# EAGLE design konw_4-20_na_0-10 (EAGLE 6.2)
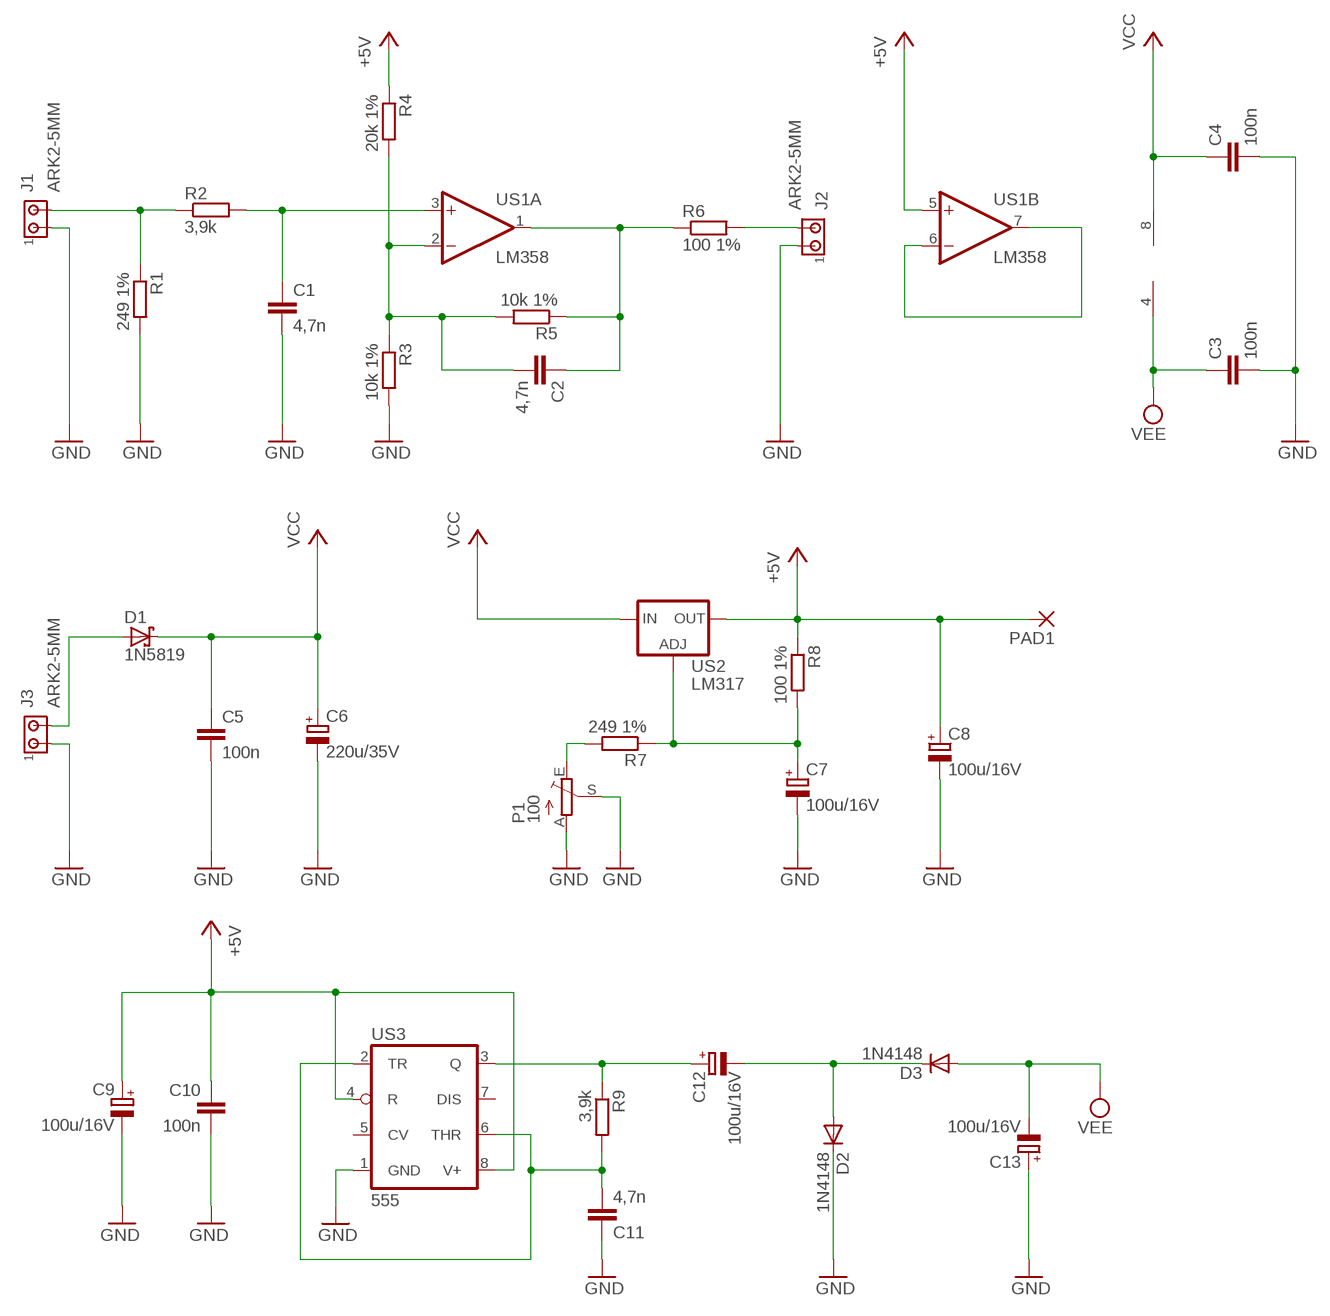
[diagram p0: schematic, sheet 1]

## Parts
C1  4,7n  C-EU050-025X075  [C050-025X075]
C2  4,7n  C-EU050-025X075  [C050-025X075]
C3  100n  C-EU050-025X075  [C050-025X075]
C4  100n  C-EU050-025X075  [C050-025X075]
C5  100n  C-EU050-025X075  [C050-025X075]
C6  220u/35V  CPOL-EUE3.5-8  [E3,5-8]
C7  100u/16V  CPOL-EUE2.5-6  [E2,5-6]
C8  100u/16V  CPOL-EUE2.5-6  [E2,5-6]
C9  100u/16V  CPOL-EUE2.5-6  [E2,5-6]
C10  100n  C-EU050-025X075  [C050-025X075]
C11  4,7n  C-EU050-025X075  [C050-025X075]
C12  100u/16V  CPOL-EUE2.5-6  [E2,5-6]
C13  100u/16V  CPOL-EUE2.5-6  [E2,5-6]
D1  1N5819  1N5819-T  [DO41-7.6]
D2  1N4148  BAT81  [DO34-7]
D3  1N4148  BAT81  [DO34-7]
J1  ARK2-5MM  [2PIN-5MM]
J2  ARK2-5MM  [2PIN-5MM]
J3  ARK2-5MM  [2PIN-5MM]
P1  100  TRIM_EU-B64Y  [B64Y]
PAD1  2,15/1,0  [2,15/1,0]
R1  249 1%  R-EU_0207/7  [0207/7]
R2  3,9k  R-EU_0207/7  [0207/7]
R3  10k 1%  R-EU_0207/7  [0207/7]
R4  20k 1%  R-EU_0207/7  [0207/7]
R5  10k 1%  R-EU_0207/7  [0207/7]
R6  100 1%  R-EU_0207/7  [0207/7]
R7  249 1%  R-EU_0207/7  [0207/7]
R8  100 1%  R-EU_0207/7  [0207/7]
R9  3,9k  R-EU_0207/7  [0207/7]
US1  LM358  LM358N  [DIL08]
US2  LM317  LM317TS  [317TS]
US3  555  LM555N  [DIL08]

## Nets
+5V: C8.+ C9.+ C10.1 PAD1.1(P) R4.1 R8.1 US1.5(B:+IN) US2.2(OUT) US3.4(R) US3.8(V+)
GND: C1.2 C3.2 C4.2 C5.2 C6.- C7.- C8.- C9.- C10.2 C11.1 C13.+ D2.C J1.P$1 J2.P$1 J3.P$1 P1.A P1.S R1.2 R3.2 US3.1(GND)
N$1: J1.P$2 R1.1 R2.1
N$2: C1.1 R2.2 US1.3(A:+IN)
N$3: C2.1 R5.1 R6.1 US1.1(A:OUT)
N$4: C2.2 R3.1 R4.2 R5.2 US1.2(A:-IN)
N$5: J2.P$2 R6.2
N$6: P1.E R7.2
N$9: US1.6(B:-IN) US1.7(B:OUT)
N$15: C12.- D2.A D3.C
N$16: C11.2 R9.2 US3.2(TR) US3.6(THR)
N$18: D1.A J3.P$2
N$19: C12.+ R9.1 US3.3(Q)
N$22: C7.+ R7.1 R8.2 US2.1(ADJ)
VCC: C4.1 C5.1 C6.+ D1.C US1.8(P:V+) US2.3(IN)
VEE: C3.1 C13.- D3.A US1.4(P:V-)
Unconnected: US3.5(CV) US3.7(DIS)

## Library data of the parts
C1-C5 C10 C11 = rcl:C-EU: CAPACITOR, European symbol
C6-C9 C12 C13 = rcl:CPOL-EU: POLARIZED CAPACITOR, European symbol
D1 = diode:1N581*: 1.0A SCHOTTKY BARRIER RECTIFIER
D2 D3 = diode:BAT81: DIODE
J1-J3 = zlacza_futrzak:ARK2: ARK 2
P1 = pot:TRIM_EU-: POTENTIOMETER
PAD1 = wirepad:2,15/1,0: THROUGH-HOLE PAD
R1-R9 = rcl:R-EU_: RESISTOR, European symbol
US1 = linear:LM358: OP AMP also LM158; LM258; LM2904 Source: http://cache.national.com/ds/LM/LM158.pdf
US2 = v-reg:LM317TS: VOLTAGE REGULATOR
US3 = linear:*555: TIMER

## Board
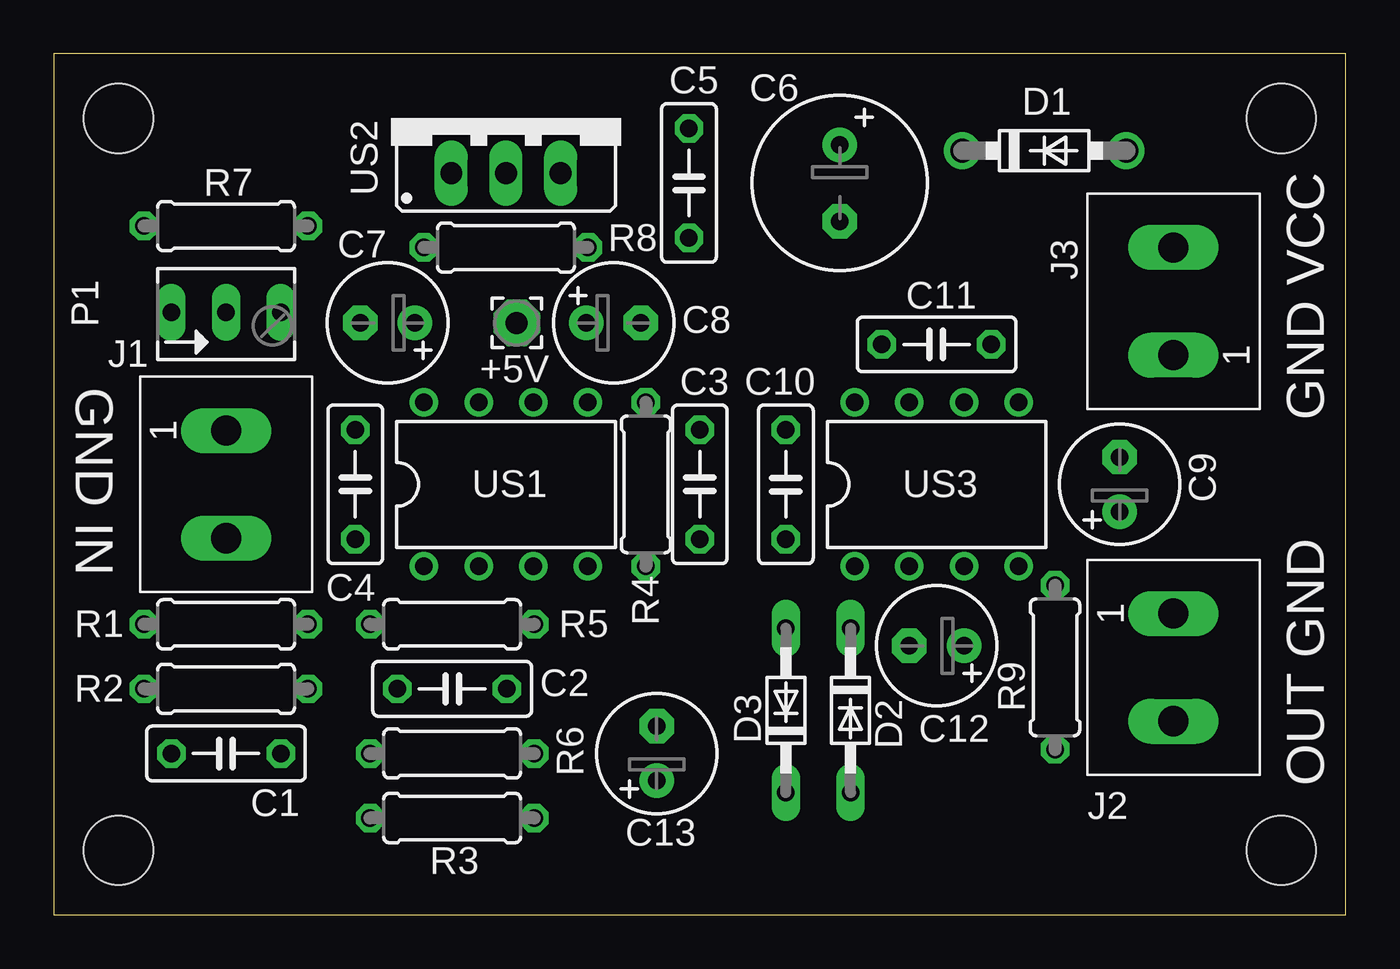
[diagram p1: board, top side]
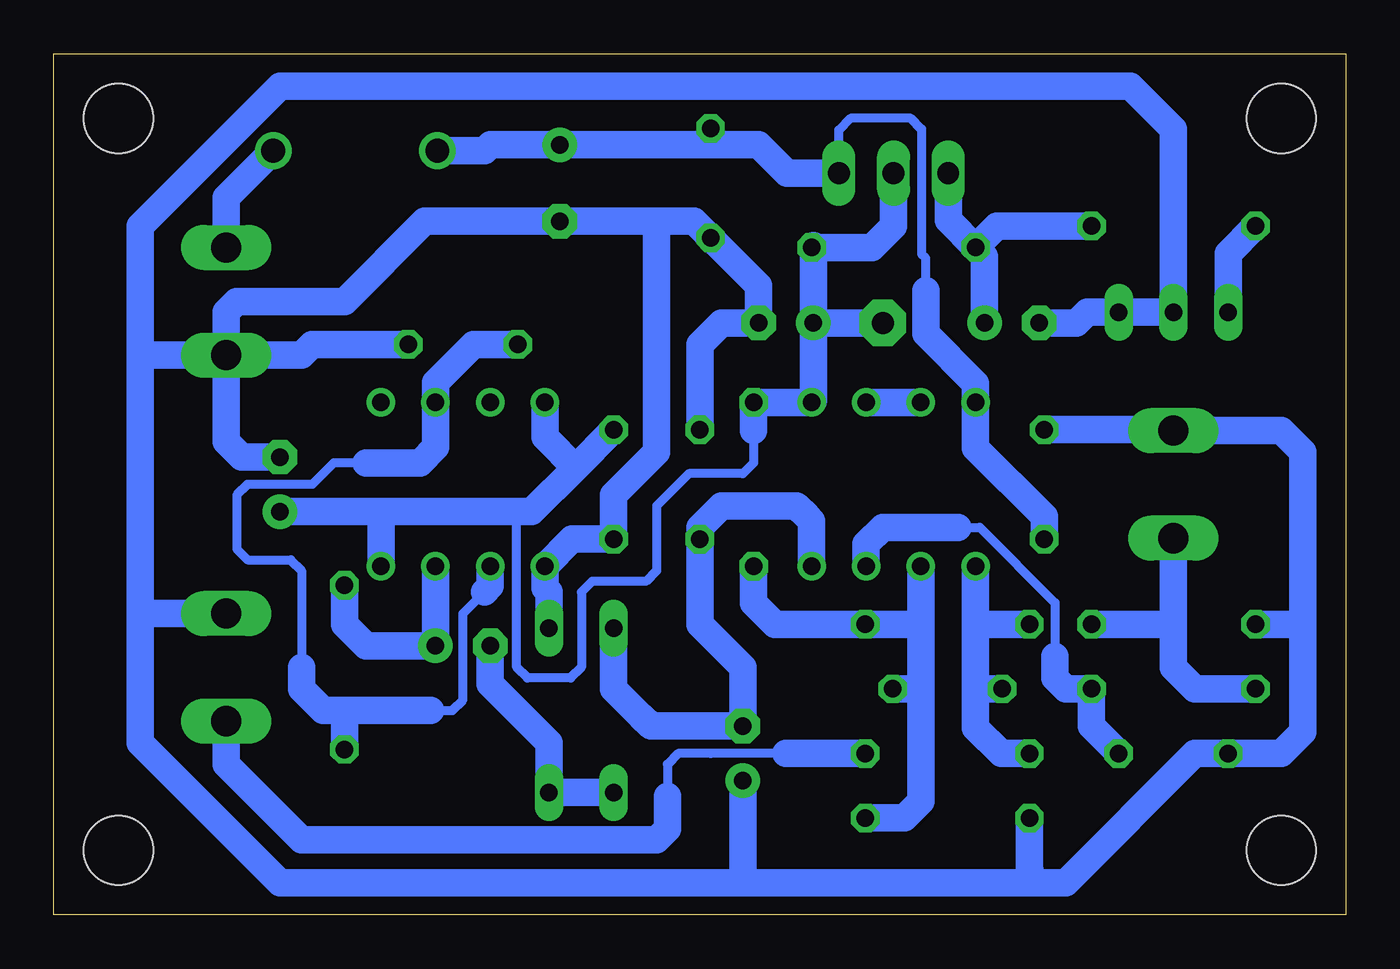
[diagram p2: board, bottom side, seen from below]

Size 60 x 40 mm. Coordinates in mm from the lower left corner, seen from the top.
Outline: 0,0 60,0 60,40 0,40 0,0
Copper layers (1*16): Top 0.035mm / dielectric 1.5mm / Bottom 0.035mm
Design rules: minimum track width 10mil, minimum drill 24mil, track to track 8mil, track to pad 8mil, pad to pad 8mil, via to via 8mil, smd to smd 8mil, copper to edge 20mil, drill to drill 8mil, minimum pad ring 10mil, minimum via ring 8mil, stop-mask expansion 4mil, vias tented up to drill 0mil, thermal gap 10mil
Holes 3.2 mm at 3,3 3,37 57,3 57,37

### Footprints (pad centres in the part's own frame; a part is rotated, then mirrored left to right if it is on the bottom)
C050-025X075 = drill 0.813 octagon: 1 -2.54,0; 2 2.54,0
E3,5-8 = drill 0.813 pad 1.6: + -1.778,0 | drill 0.813 pad 1.6 octagon: - 1.778,0
E2,5-6 = drill 0.813 pad 1.6: + -1.27,0 | drill 0.813 pad 1.6 octagon: - 1.27,0
DO41-7.6 = drill 1.1 pad 1.7: A 3.81,0; C -3.81,0
DO34-7 = drill 0.813 long: A 3.81,0; C -3.81,0
2PIN-5MM = drill 1.4 long: P$1 -2.5,0; P$2 2.5,0
B64Y = drill 0.813 long: A 2.54,0; E -2.54,0; S 0,0
2,15/1,0 = drill 1.016 pad 2.159 octagon: 1 0,0
0207/7 = drill 0.813 octagon: 1 -3.81,0; 2 3.81,0
DIL08 = drill 0.813 pad 1.27: 1 -3.81,-3.81; 2 -1.27,-3.81; 3 1.27,-3.81; 4 3.81,-3.81; 5 3.81,3.81; 6 1.27,3.81; 7 -1.27,3.81; 8 -3.81,3.81
317TS = drill 1.016 long: 1 -2.54,-2.54; 2 0,-2.54; 3 2.54,-2.54

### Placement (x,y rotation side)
C1  8,7.5 180 top
C2  18.5,10.5 0 top
C3  30,20 90 top
C4  14,20 90 top
C5  29.5,34 270 top
C6  36.5,34 270 top
C7  15.5,27.5 180 top
C8  26,27.5 0 top
C9  49.5,20 90 top
C10  34,20 270 top
C11  41,26.5 180 top
C12  41,12.5 180 top
C13  28,7.5 90 top
D1  46,35.5 0 top
D2  37,9.5 270 top
D3  34,9.5 90 top
J1  8,20 270 top
J2  52,11.5 270 top
J3  52,28.5 90 top
P1  8,28 0 top
PAD1  21.5,27.5 0 top
R1  8,13.5 180 top
R2  8,10.5 0 top
R3  18.5,4.5 180 top
R4  27.5,20 270 top
R5  18.5,13.5 0 top
R6  18.5,7.5 0 top
R7  8,32 180 top
R8  21,31 180 top
R9  46.5,11.5 270 top
US1  21,20 0 top
US2  21,37 0 top
US3  41,20 0 top

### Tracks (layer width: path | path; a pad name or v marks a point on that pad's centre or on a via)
+5V
  Bottom 0.406: 27.5,22.5 27.5,21 28,20.5 30.5,20.5 32,19 32,16 32.5,15.5 35,15.5 35.5,15 35.5,11.5 36,11 38,11 38.5,11.5 38.5,18.73
  Bottom 1.27: C9.+ 45,18.73 | 45,18.73 38.5,18.73 37.81,18.73 35.77,20.77 | 35.77,20.77 C10.1 | US3.8 37.19,22.19 35.77,20.77 | US3.4 44.81,18.54 45,18.73 | C8.+ 24.73,23.89 US1.5 R4.1 27.5,22.5 | C8.+ 24.73,31.08 R8.1 22,31 21,32 US2.2 | PAD1.1 C8.+
GND
  Bottom 1.27: 2,13.5 2,21.5 3,22.5 J1.P$1 8.04,22.54 C4.2 | 2,13.5 2,8.5 3,7.5 C1.2 7,7.5 13,1.5 14.5,1.5 | R1.2 2,13.5 | 14.5,1.5 28,1.5 | 28,1.5 49.5,1.5 56,8 56,14 | 56,14 56,26 | J3.P$1 56,26 | J2.P$1 56,14 | R3.2 14.69,2.19 14.5,1.5 | C13.+ 28,1.5 | D2.C 37,15 37.19,15.19 US3.1 35.92,17.46 C10.2 34,19.5 32,21.5 32,32.22 | 56,26 56,32 49.5,38.5 10,38.5 8,36.5 P1.S P1.A 12,28 12.5,27.5 C7.- | C11.1 48,26.5 48.5,26 J3.P$1 | J3.P$1 52,22 51.27,21.27 C9.- | J3.P$1 52,28 51.5,28.5 46.5,28.5 42.78,32.22 C6.- 32,32.22 | 32,32.22 30.26,32.22 C5.2 27.27,29.23 C8.- 29,27.5 30,26.5 C3.2
N$1
  Bottom 1.27: J1.P$2 8,13.5 | 8,13.5 8,11.5 7,10.5 R2.1 | R1.1 8,13.5
N$2
  Bottom 0.406: 18,18 17,18 13.5,14.5 13.5,12
  Bottom 1.27: C1.1 11.81,8.77 R2.2 13,10.5 13.5,11 13.5,12 | US1.3 22.27,17.23 21.5,18 18,18
N$3
  Bottom 1.27: US1.1 17.19,13.5 | 17.19,13.5 17.19,10.5 | 17.19,10.5 17.19,8.69 16,7.5 R6.1 | C2.1 17.19,10.5 | R5.1 17.19,13.5
N$4
  Bottom 1.27: US1.2 19.73,13.5 | 19.73,13.5 19.73,10.5 | 19.73,10.5 19.73,5.27 20.5,4.5 R3.1 | C2.2 19.73,10.5 | 19.73,13.5 R5.2 26.5,13.5 27.5,14.5 R4.2
N$5
  Bottom 0.406: 26,7.5 29.5,7.5 31,7.5 31.5,7 31.5,5.5
  Bottom 1.27: R6.2 26,7.5 | 31.5,5.5 31.5,4 32,3.5 48.5,3.5 52,7 J2.P$2
N$6
  Bottom 1.27: P1.E 5.46,30.73 R7.2
N$9
  Bottom 1.27: US1.7 US1.6
N$15
  Bottom 1.27: D3.C D2.A 37,8 39.73,10.73 C12.-
N$16
  Bottom 0.406: 45.5,21 47,21 48,20 51,20 51.5,19.5 51.5,17 51,16.5 49,16.5 48.5,16 48.5,11.5 | 42.5,9.5 41.5,9.5 41,10 41,14 40,15
  Bottom 1.27: 45.5,21 43,21 42.27,21.73 US3.6 42.27,24.73 40.5,26.5 C11.2 | 48.5,11.5 48.5,10.5 47.5,9.5 46.5,9.5 | 46.5,9.5 42.5,9.5 | US3.2 39.73,15.27 40,15 | R9.2 46.5,9.5
N$18
  Bottom 1.27: J3.P$2 52,33.31 D1.A
N$19
  Bottom 1.27: US3.3 C12.+ 45.5,12.5 46.5,13.5 R9.1
N$22
  Bottom 1.27: US2.1 18.46,32.27 R8.2 | C7.+ 16.77,30.58 R8.2 | R7.1 16.19,32 R8.2
VCC
  Bottom 0.406: 19.5,29 19.5,30.5 19.7,30.7 19.7,36.5 20.2,37 23,37 23.54,36.46 US2.3
  Bottom 1.27: C4.1 14,18.5 17.19,21.69 US1.8 17.19,24.69 19.5,27 19.5,29 | D1.C 40,35.5 39.72,35.78 C6.+ 29.5,35.78 | 29.5,35.78 27.28,35.78 25.96,34.46 US2.3 | C5.1 29.5,35.78
VEE
  Bottom 1.27: D3.A 34,10.5 33,9.5 32.75,9.25 | 32.75,9.25 32.5,9 | 32.75,9.25 32.27,8.77 C13.- 28,11.5 30,13.5 C3.1 30,18 29,19 25.5,19 25,18.5 24.81,18.31 US1.4

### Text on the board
tPlace: +5V | GND IN | GND VCC | OUT GND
